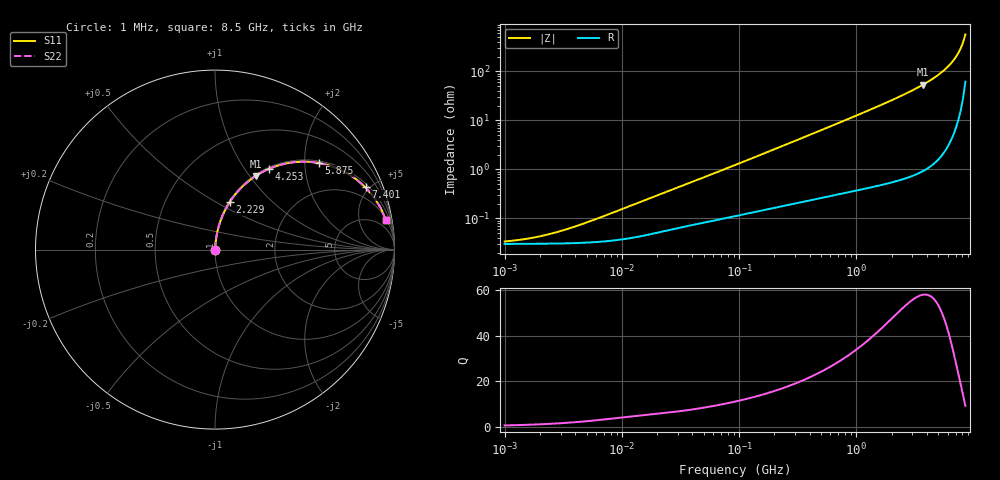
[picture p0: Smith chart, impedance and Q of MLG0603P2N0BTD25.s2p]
! S-Parameter Data Generated by TDK Corporation
! Copyright(C) 2025 TDK Corporation.
! All Rights Reserved.
! TDK P/N: MLG0603P2N0BTD25 (SMD / SMT Inductor (Coil))
! Property: L=2nH at 500MHz
! Size(LxWxT): 0.6x0.3x0.3mm
! Model Type: s2p (Touchstone File Format Version 1.0)
! Frequency: DC=Yes Start=1MHz Stop=8500MHz 198points Log-sweep
! Model Generated on Feb. 6, 2025
! Terms and conditions regarding TDK Simulation Models:
! 1)This simulation model is being provided solely for informational
!  purposes. Please refer to the specifications of the products in
!  terms of detailed characteristics of such products.
! 2)In no event shall TDK Corporation of any of its subsidiaries be
!  liable for any loss or damage arising, directly or indirectly,
!  from any information contained in this simulation model, including,
!  but not limited to loss or damages arising from any inaccuracies,
!  omissions or errors in connection with such information.
! 3)Any and all copyrights on this simulation model are owned by
!  TDK Corporation.  Duplication or redistribution of this simulation
!  model without prior written permission from TDK Corporation
!  is prohibited.
! 4)This simulation model is subject to any modification or change
!  without any prior notice.
! 5)Neither TDK Corporation nor any of its subsidiaries shall make any
!  warranty, express or implied, including but not limited to the
!  correctness, implied warranties of merchantability and fitness for
!  a particular purpose with respect to this simulation models.
! 6)The use of this simulation model shall be deemed to have consented
!  to the terms and conditions hereof.
! Port Assignments:
!  1 ---@@@--- 2
! Applicable Conditions:
!  Temperature = 25 degC
!  DC Bias Current = 0 A
!  Small Signal Operation
# Hz S MA R 50
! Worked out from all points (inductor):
!   197 points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, 1 MHz to 8.5 GHz, reference 50 ohm
!   read as one part in series: L = 2.4 nH near 6.637 MHz
!   highest Q = 58.1 at 3.703 GHz (marker M1), where L = 2.3 nH
!   S11 on the Smith chart (normalised r, x): 1 MHz: 1.00, +0.00; 2.229 GHz: 1.01, +0.58; 4.253 GHz: 1.02, +1.31; 5.875 GHz: 1.05, +2.35; 7.401 GHz: 1.20, +4.74; 8.5 GHz: 2, +11
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1000000  0.0003371 26.9  0.9997 -0.0  0.9997 -0.0  0.0003371 26.9
1446720  0.0003735 36.1  0.9997 -0.0  0.9997 -0.0  0.0003735 36.1
2092998  0.00044 46.4  0.9997 -0.0  0.9997 -0.0  0.00044 46.4
3027982  0.0005537 56.3  0.9997 -0.0  0.9997 -0.0  0.0005537 56.3
4587603  0.0007647 65.5  0.9997 -0.0  0.9997 -0.0  0.0007647 65.5
2.10461e7  0.003081 80.1  0.9995 -0.2  0.9995 -0.2  0.003081 80.1
9.219544e7  0.01222 84.1  0.9988 -0.7  0.9988 -0.7  0.01222 84.1
4.229561e8  0.05316 84.4  0.9962 -3.0  0.9962 -3.0  0.05316 84.4
9.708683e8  0.1203 81.4  0.9891 -6.9  0.9891 -6.9  0.1203 81.4
1.404574e9  0.1737 78.6  0.9805 -10.0  0.9805 -10.0  0.1737 78.6
1.940355e9  0.2404 74.9  0.9656 -13.9  0.9656 -13.9  0.2404 74.9
2.228565e9  0.2768 72.8  0.9554 -16.1  0.9554 -16.1  0.2768 72.8
2.939772e9  0.3682 67.4  0.9231 -21.6  0.9231 -21.6  0.3682 67.4
3.703002e9  0.4688 61.1  0.8753 -28.0  0.8753 -28.0  0.4688 61.1
4.253027e9  0.5425 56.2  0.8307 -32.8  0.8307 -32.8  0.5425 56.2
5.115526e9  0.6573 47.8  0.7412 -41.1  0.7412 -41.1  0.6573 47.8
5.87536e9  0.7534 39.8  0.6408 -48.9  0.6408 -48.9  0.7534 39.8
6.748056e9  0.8502 30.0  0.501 -58.2  0.501 -58.2  0.8502 30.0
7.400733e9  0.9076 22.5  0.3827 -65.1  0.3827 -65.1  0.9076 22.5
7.750377e9  0.9318 18.4  0.3161 -68.5  0.3161 -68.5  0.9318 18.4
8.116539e9  0.9518 14.2  0.2453 -71.7  0.2453 -71.7  0.9518 14.2
8.5e9  0.9669 9.8  0.1709 -74.0  0.1709 -74.0  0.9669 9.8
